FUNCTION FC 15 : VOID
TITLE =I CHECK TRANSMISSION RECIPE
AUTHOR : Esposito
FAMILY : EGAL_SRL
NAME : BIT_OP37
VERSION : 0.1

BEGIN
NETWORK
TITLE =

      L     S5T#10S;
      L     T     60;
      <>I   ;
      L     S5T#10S;
      SE    T     60;
NETWORK
TITLE =CONTROLLO FINE TRASMISSIONE RICETTA DA OP37 A PLC

      L     DB11.DBW    2;
      L     9;
      ==I   ;
      =     M    120.0;
NETWORK
TITLE =CONFERMA DI RICEZIONE OK RICETTA DA PLC

      O     M    120.0;
      O     T     61;
      FP    M    120.1;
      =     M    120.2;
      UN    M    120.2;
      SPB   M001;

      L     4;
      T     DB11.DBW    2;
M001: NOP   0;
NETWORK
TITLE =
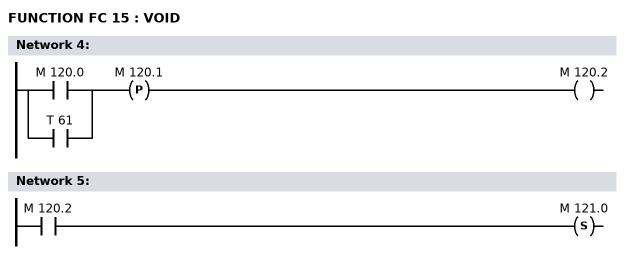
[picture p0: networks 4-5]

      U(    ;
      O     M    120.0;
      O     T     61;
      )     ;
      FP    M    120.1;
      =     M    120.2;
NETWORK
TITLE =

      U     M    120.2;
      S     M    121.0;

END_FUNCTION

